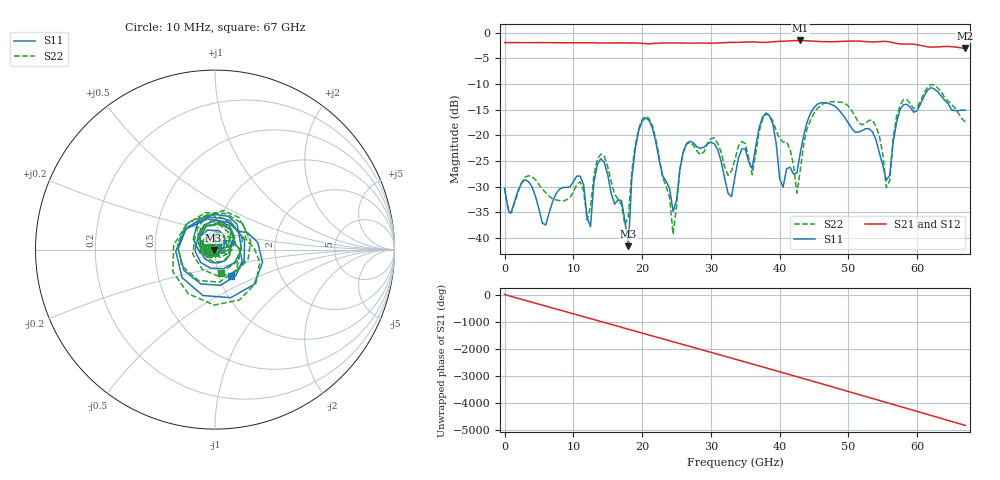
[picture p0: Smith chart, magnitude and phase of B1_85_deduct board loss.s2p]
!Keysight Technologies,N5247B,MY61255065,A.16.20.04
!Date: Sunday, September 03, 2023 21:45:05
!Correction: S11(C  2-Port  )
!S21(C  2-Port  )
!S12(C  2-Port  )
!S22(C  2-Port  )
!S2P File: Measurements: S11, S21, S12, S22:
!Deduct Board Loss
# Hz S  dB  R 50
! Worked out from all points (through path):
!   142 points, 10 MHz to 67 GHz, reference 50 ohm
!   highest |S21| = -1.54 dB at 43 GHz (marker M1); lowest = -3.0 dB at 67 GHz (marker M2)
!   lowest |S11| = -41.6 dB at 18 GHz (marker M3), VSWR 1.02, Z = 49.2 - j0.215 ohm
!   |S11| at or under -10 dB: start of sweep to end of sweep
!   |S22| runs from -39.2 to -10.1 dB; largest |S21 - S12| = 0.0025
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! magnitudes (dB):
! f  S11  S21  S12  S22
! 10 MHz  -30.3  -1.9  -1.9  -30.4
! 6 GHz  -37.5  -2.0  -2.0  -31.2
! 11.5 GHz  -29.7  -2.0  -2.0  -30.8
! 12.5 GHz  -37.8  -2.0  -2.0  -33.9
! 14.5 GHz  -25.3  -2.0  -2.0  -24.1
! 18 GHz  -41.6  -2.0  -2.0  -35.7
! 18.5 GHz  -28.4  -2.0  -2.0  -27.1
! 20 GHz  -17.2  -2.1  -2.1  -17.0
! 22.5 GHz  -25.0  -2.1  -2.1  -24.4
! 24.5 GHz  -34.8  -2.0  -2.0  -39.2
! 26.5 GHz  -21.5  -2.1  -2.1  -21.7
! 33 GHz  -32.0  -1.9  -1.9  -26.9
! 34 GHz  -24.4  -1.9  -1.9  -22.1
! 36 GHz  -26.5  -1.8  -1.8  -27.6
! 38.5 GHz  -16.1  -1.8  -1.8  -16.1
! 40.5 GHz  -30.1  -1.7  -1.7  -21.3
! 43 GHz  -23.4  -1.5  -1.5  -26.7
! 45 GHz  -14.6  -1.7  -1.7  -15.7
! 53.5 GHz  -19.3  -1.8  -1.8  -17.1
! 56 GHz  -27.8  -1.8  -1.8  -28.8
! 58 GHz  -14.0  -2.2  -2.2  -13.1
! 67 GHz  -15.1  -3.0  -3.0  -17.4
